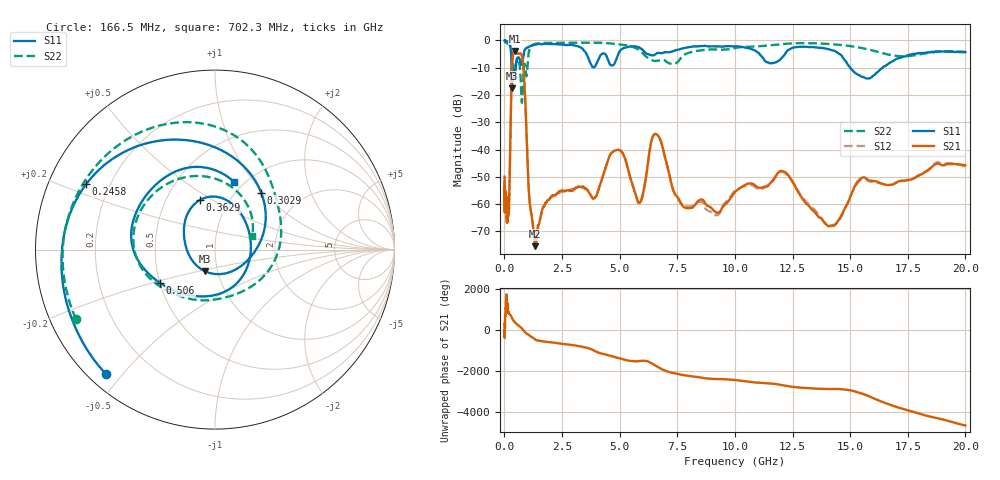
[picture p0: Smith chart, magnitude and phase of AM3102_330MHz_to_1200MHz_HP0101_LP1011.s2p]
! Date/Time: Tue, Sep 11, 2018 5:14 PM
! Network Analyzer: Agilent Technologies E8362B Rev: A.07.50.63
! Sweep from 0.010 to 20.000 GHz, 1601 Points, Sweep Type: LOG
! Power Supply: 4.949 V, 0.001 A
# Hz S DB R 50
!freq MagS11 AngS11 MagS21 AngS21 MagS12 AngS12 MagS22 AngS22
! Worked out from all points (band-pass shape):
!   1601 points, 10 MHz to 20 GHz, reference 50 ohm
!   highest |S21| = -3.81 dB at 469 MHz (marker M1); lowest = -75.4 dB at 1.34 GHz (marker M2)
!   |S21| within 3 dB of the highest: 350.7 MHz to 787.4 MHz (436.6 MHz wide, 76.7 % of centre)
!   lowest |S11| = -17.5 dB at 331.5 MHz (marker M3), VSWR 1.31, Z = 43.4 - j10.7 ohm
!   |S11| at or under -10 dB: 309.6 MHz to 493.4 MHz (183.8 MHz wide, 45.8 % of centre); 15 GHz to 16.4 GHz (1.4 GHz wide, 8.91 % of centre)
!   |S22| runs from -22.8 to -0.3 dB; largest |S21 - S12| = 0.011
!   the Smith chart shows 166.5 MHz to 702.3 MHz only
!   S11 on the Smith chart (normalised r, x): 166.5 MHz: 0.05, -0.45; 245.8 MHz: 0.11, +0.24; 302.9 MHz: 1.28, +0.97; 362.9 MHz: 0.73, +0.44; 506 MHz: 0.50, -0.21; 702.3 MHz: 0.90, +0.80
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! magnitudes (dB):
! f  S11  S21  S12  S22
! 10 MHz  0.0  -49.9  -54.7  -0.3
! 35.55 MHz  0.0  -58.8  -58.4  -0.5
! 126.4 MHz  -0.4  -65.2  -63.4  -1.1
! 166.5 MHz  -0.7  -63.0  -63.4  -1.3
! 245.8 MHz  -1.9  -42.7  -42.6  -1.8
! 302.9 MHz  -7.8  -16.9  -17.0  -3.5
! 331.5 MHz  -17.5  -9.1  -9.1  -6.2
! 362.9 MHz  -10.8  -6.0  -6.1  -8.5
! 447.2 MHz  -13.0  -3.8  -3.9  -10.7
! 469 MHz  -11.8  -3.8  -3.8  -9.9
! 506 MHz  -8.9  -4.0  -4.1  -8.2
! 702.3 MHz  -8.2  -4.8  -4.8  -13.1
! 1.34 GHz  -1.5  -75.4  -72.8  -1.2
! 1.59 GHz  -1.4  -63.9  -64.2  -1.0
! 3.902 GHz  -9.8  -57.8  -57.7  -0.8
! 4.855 GHz  -6.9  -40.2  -40.3  -1.3
! 5.652 GHz  -2.2  -55.2  -55.5  -2.6
! 6.58 GHz  -4.9  -34.3  -34.4  -7.5
! 9.047 GHz  -2.2  -62.0  -63.3  -3.3
! 12.09 GHz  -5.9  -47.9  -48.3  -1.3
! 14.14 GHz  -3.4  -68.1  -67.8  -1.3
! 20 GHz  -4.3  -45.8  -46.2  -4.1
